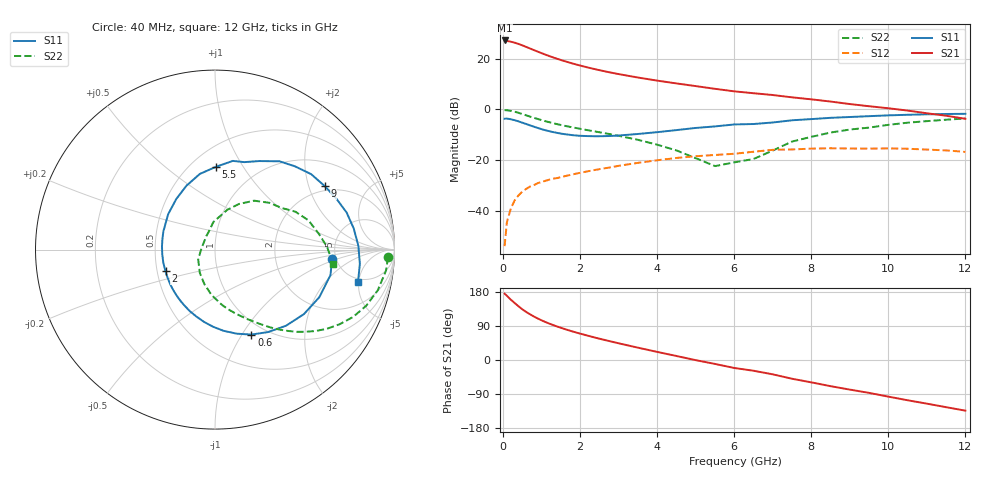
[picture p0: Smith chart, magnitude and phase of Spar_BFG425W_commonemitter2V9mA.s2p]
! Filename: 29bfg425.001
! BFG425W Field C1
! V1=8.439E-001V,V2=2.000E+000V, I1=1.211E-004A, I2=8.990E-003A
# GHz  S  MA  R 50
!  S11  S21  S12  S22
!Freq(GHz)  Mag  Ang  Mag  Ang  Mag  Ang  Mag  Ang
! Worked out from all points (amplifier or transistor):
!   44 points, 40 MHz to 12 GHz, reference 50 ohm
!   highest |S21| = 27.2 dB at 40 MHz (marker M1)
!   |S21| within 3 dB of that: start of sweep to 672.1 MHz
!   unconditionally stable (mu >= 1): 1.951 GHz to end of sweep
!   at 700 MHz: K = 0.50, MSG = 27.2 dB, |S12| = -30.5 dB
!   at 2.4 GHz: K = 1.09, MAG = 18.0 dB, |S12| = -23.9 dB
!   at 12 GHz: K = 1.40, MAG = 2.8 dB, |S12| = -16.8 dB
!   S11 on the Smith chart (normalised r, x): 40 MHz: 4.60, -0.89; 600 MHz: 0.85, -1.10; 2 GHz: 0.55, -0.15; 5.5 GHz: 0.65, +0.77; 9 GHz: 1.82, +2.57; 12 GHz: 4.51, -4.89
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0.04  0.654 -4.8  22.89 175.1  0.002 78.6  0.965 -2.6
0.2  0.639 -24.5  21.66 159.3  0.011 77.2  0.935 -14.0
0.3  0.612 -36.0  20.69 150.4  0.016 71.9  0.899 -20.3
0.4  0.58 -47.0  19.55 141.8  0.02 66.7  0.856 -26.0
0.5  0.546 -57.3  18.34 133.7  0.024 62.8  0.809 -31.0
0.6  0.515 -66.8  17.07 126.8  0.027 59.5  0.764 -35.3
0.8  0.455 -84.0  14.79 114.8  0.032 54.2  0.681 -42.2
0.9  0.43 -91.5  13.78 109.5  0.035 52.3  0.646 -45.2
1  0.407 -98.8  12.85 104.7  0.037 50.6  0.613 -47.8
1.2  0.371 -112.1  11.27 96.0  0.041 48.0  0.558 -52.3
1.6  0.324 -135.9  8.927 81.7  0.048 44.5  0.474 -59.8
2  0.301 -156.4  7.32 69.6  0.056 41.4  0.414 -66.6
2.2  0.297 -165.9  6.703 64.1  0.06 39.8  0.388 -70.1
3  0.305 160.6  4.967 44.1  0.077 32.3  0.301 -84.5
3.5  0.327 143.0  4.25 32.5  0.088 26.7  0.251 -94.9
4.5  0.39 114.0  3.252 10.6  0.11 13.4  0.155 -123.1
5.5  0.461 89.4  2.543 -10.4  0.126 -1.2  0.076 175.3
6.5  0.514 71.4  2.083 -28.3  0.146 -12.4  0.105 109.4
8.5  0.681 38.1  1.427 -69.1  0.171 -48.7  0.349 51.4
9  0.707 29.9  1.274 -78.1  0.169 -56.8  0.4 40.7
10.5  0.782 8.6  0.947 -106.2  0.167 -83.5  0.546 17.3
12  0.817 -12.7  0.652 -133.6  0.145 -113.2  0.662 -6.8
